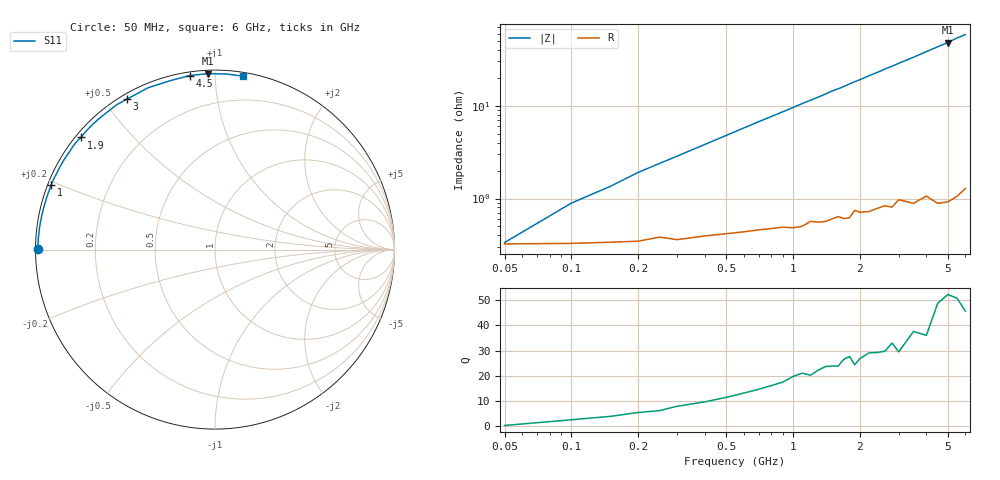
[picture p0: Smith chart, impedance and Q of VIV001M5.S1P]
! Infineon Technologies  Discrete & RF Semiconductors
! BB 804
! Si Tuning Diode in SOT23
! VR =
! S-Parameters:  July  1999
# GHz  S  MA  R  50
!  f  S11
! GHz  MAG  ANG
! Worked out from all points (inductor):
!   34 points, 50 MHz to 6 GHz, reference 50 ohm
!   read as one part to ground: L = 1.49 nH near 150 MHz
!   highest Q = 50.8 at 5 GHz (marker M1), where L = 1.53 nH
!   S11 on the Smith chart (normalised r, x): 50 MHz: 0.01, +0.00; 1 GHz: 0.01, +0.19; 1.9 GHz: 0.01, +0.36; 3 GHz: 0.02, +0.57; 4.5 GHz: 0.02, +0.86; 6 GHz: 0.03, +1.17
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0.05  0.9871 179.8
0.1  0.987 178.1
0.15  0.9866 177.0
0.2  0.9863 175.7
0.3  0.9857 173.5
0.5  0.9836 169.1
0.8  0.9816 162.6
1  0.9815 158.4
1.1  0.981 156.2
1.3  0.9792 152.2
1.4  0.9791 150.1
1.5  0.978 147.9
1.6  0.9769 146.1
1.7  0.9782 144.2
1.8  0.978 142.1
1.9  0.974 140.1
2  0.9754 138.3
2.2  0.9757 134.4
2.4  0.9745 130.9
2.6  0.9735 127.1
2.8  0.9752 123.9
3  0.9712 120.4
3.5  0.9757 112.6
4  0.9736 105.1
4.5  0.9799 98.3
5  0.9811 92.3
5.5  0.9806 85.9
6  0.9786 80.9
